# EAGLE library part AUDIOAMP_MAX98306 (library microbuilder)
MAX98306 3.7W Stereo Audio Amp - TDFN14 3.7W @ 3 ohm, 2.6-5.5V supply, 6-18dB selectable gain
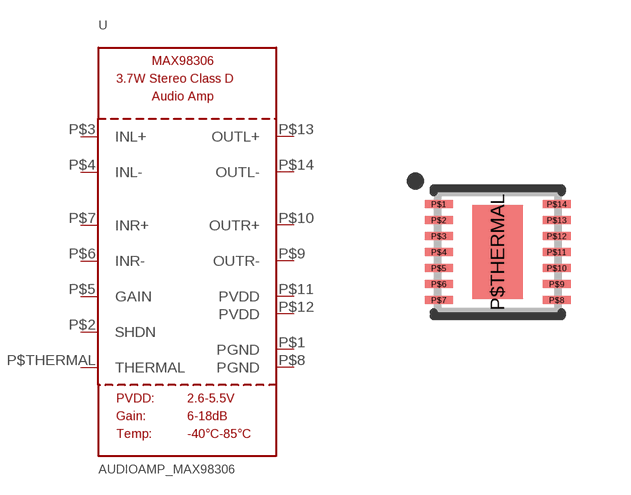
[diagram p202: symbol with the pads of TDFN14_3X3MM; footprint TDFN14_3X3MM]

Designator prefix U

## AUDIOAMP_MAX98306  [TDFN14_3X3MM]
P$1  PGND  pwr
P$2  SHDN  in
P$3  INL+  in
P$4  INL-  in
P$5  GAIN  in
P$6  INR-  in
P$7  INR+  in
P$8  PGND  pwr
P$9  OUTR-  out
P$10  OUTR+  out
P$11  PVDD  pwr
P$12  PVDD  pwr
P$13  OUTL+  out
P$14  OUTL-  out
P$THERMAL  THERMAL  pwr

## Footprint TDFN14_3X3MM (pad centres in mm)
TDFN 14 3x3x0.75mm Source: http://datasheets.maxim-ic.com/en/ds/MAX98306.pdf Based on recommendtions in: http://www.freescale.com/files/sensors/doc/data_sheet/MAG3110.pdf
smd 0.7 x 0.2: P$1 -1.475,1.2; P$2 -1.475,0.8; P$3 -1.475,0.4; P$4 -1.475,0; P$5 -1.475,-0.4; P$6 -1.475,-0.8; P$7 -1.475,-1.2; P$8 1.475,-1.2; P$9 1.475,-0.8; P$10 1.475,-0.4; P$11 1.475,0; P$12 1.475,0.4; P$13 1.475,0.8; P$14 1.475,1.2
smd 1.27 x 2.35: P$THERMAL 0,0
